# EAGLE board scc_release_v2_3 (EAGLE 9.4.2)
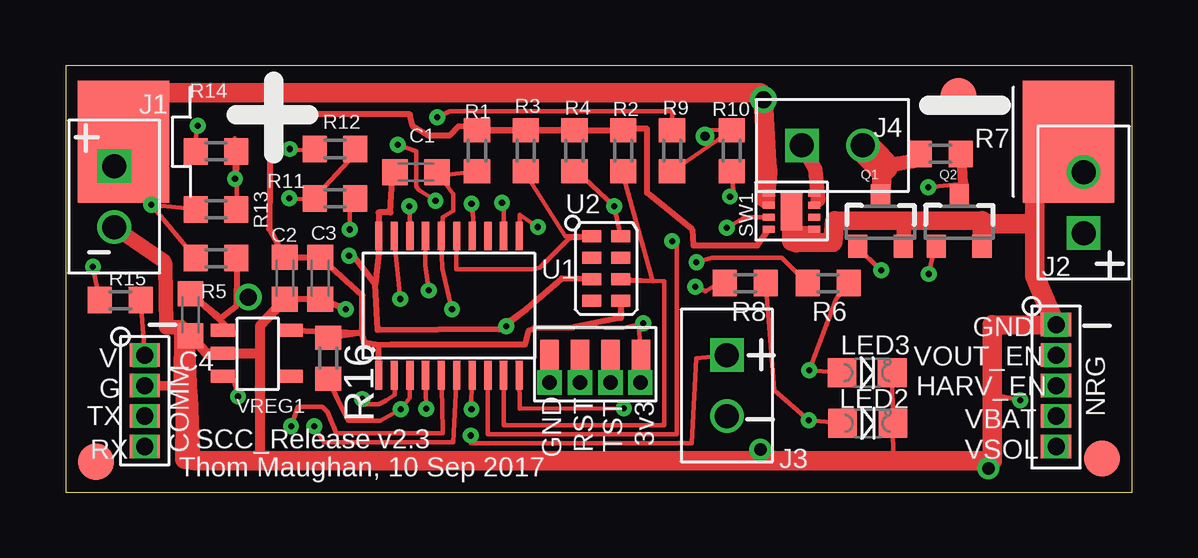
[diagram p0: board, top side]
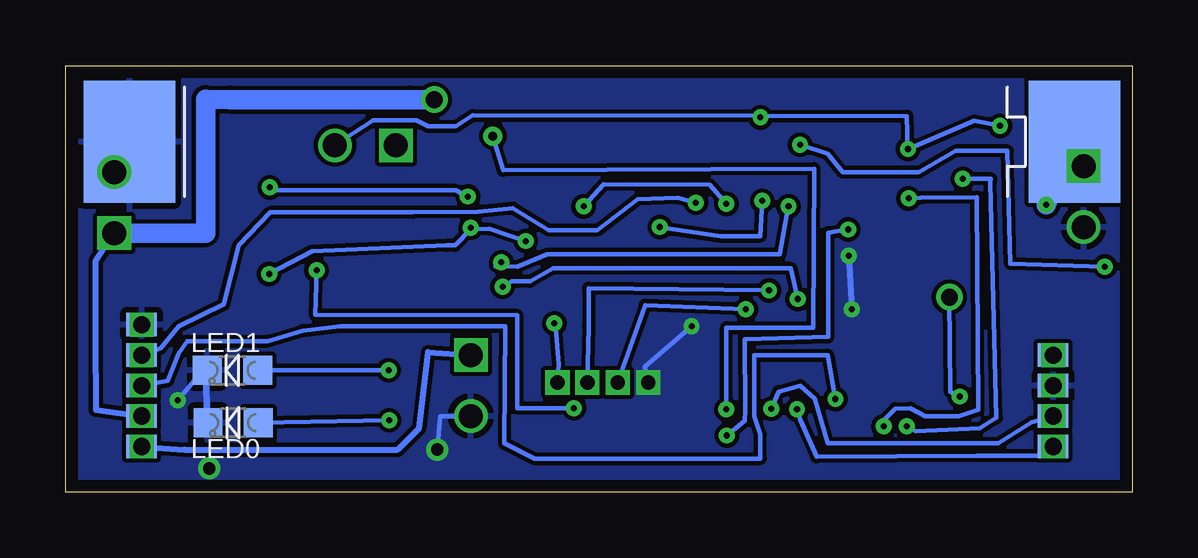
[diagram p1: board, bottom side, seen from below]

Size 44.45 x 17.78 mm. Coordinates in mm from the lower left corner, seen from the top.
Outline: 0,0 44.45,0 44.45,17.78 0,17.78 0,0
Copper layers (1*16): Top 0.035mm / dielectric 1.5mm / Bottom 0.035mm
Design rules "default *": minimum track width 7mil, minimum drill 8mil, track to track 7mil, track to pad 7mil, pad to pad 7mil, via to via 7mil, smd to smd 7mil, copper to edge 20mil, drill to drill 7mil, minimum pad ring 5mil, minimum via ring 8mil, stop-mask expansion 4mil, vias tented up to drill 11mil, thermal gap 10mil

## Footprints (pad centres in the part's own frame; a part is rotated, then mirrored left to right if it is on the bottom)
BAT_10440 = smd 3.81 x 5.08: P$1 0.508,4.572; P$2 39.878,4.572
C0603K = smd 1.05 x 1.08: 1 -0.875,0; 2 0.875,0
CON_1X4_050 = drill 0.711 pad 0.965 square: P$1 0,1.905; P$2 0,0.635; P$3 0,-0.635; P$4 0,-1.905 | smd 1.27 x 0.965: P$5 0,1.905; P$6 0,0.635; P$7 0,-0.635; P$8 0,-1.905 | smd 1.27 x 0.965 bottom: P$9 0,1.905; P$10 0,0.635; P$11 0,-0.635; P$12 0,-1.905
EMU_MSP_SPYBYWIRE_4_050 = smd 1.524 x 0.762: P1_3V3 0,1.905; P2_TST 0,0.635; P3_RST* 0,-0.635; P4_GND 0,-1.905
CON_1X2_0_1 = drill 1 square: P$1 0,1.27 | drill 1: P$2 0,-1.27
FIDUCIAL-1.5X3 = smd 1.5 x 1.5: 1 0,0
CHIPLED_0805 = smd 1.2 x 1.2: A 0,-1.05; C 0,1.05
CON_1X5_050 = drill 0.711 pad 0.965 square: P$1 0,2.54; P$2 0,1.27; P$3 0,0; P$4 0,-1.27; P$5 0,-2.54 | smd 1.27 x 0.965: P$6 0,2.54; P$7 0,1.27; P$8 0,0; P$9 0,-1.27; P$10 0,-2.54 | smd 1.27 x 0.965 bottom: P$11 0,2.54; P$12 0,1.27; P$13 0,0; P$14 0,-1.27; P$15 0,-2.54
SOT23-3 = smd 0.8 x 0.95: 1 -0.95,-1; 2 0.95,-1; 3 0,1.1
R0603 = smd 1 x 1.1: 1 -0.85,0; 2 0.85,0
TI_WSON8 = smd 0.5 x 0.28: P$1 -0.95,0.75; P$2 -0.95,0.25; P$3 -0.95,-0.25; P$4 -0.95,-0.75; P$5 0.95,-0.75; P$6 0.95,-0.25; P$7 0.95,0.25; P$8 0.95,0.75 | smd 0.9 x 1.6: P$9 0,0
PW20 = smd 0.3 x 1.2: 1 -2.925,-2.9; 2 -2.275,-2.9; 3 -1.625,-2.9; 4 -0.975,-2.9; 5 -0.325,-2.9; 6 0.325,-2.9; 7 0.975,-2.9; 8 1.625,-2.9; 9 2.275,-2.9; 10 2.925,-2.9; 11 2.925,2.9; 12 2.275,2.9; 13 1.625,2.9; 14 0.975,2.9; 15 0.325,2.9; 16 -0.325,2.9; 17 -0.975,2.9; 18 -1.625,2.9; 19 -2.275,2.9; 20 -2.925,2.9
M41T62_PKG = smd 0.8 x 0.5: P$1 -0.6,1.35; P$2 -0.6,0.45; P$3 -0.6,-0.45; P$4 -0.6,-1.35; P$5 0.6,-1.35; P$6 0.6,-0.45; P$7 0.6,0.45; P$8 0.6,1.35
SOT23-5 = smd 1 x 0.54: P$1 -1.431,0.95; P$2 -1.431,0; P$3 -1.431,-0.95; P$4 1.419,-0.95; P$5 1.419,0.95

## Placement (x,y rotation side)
BAT1  [BAT_10440]  42.29,10.03 0 bottom
BAT2  [BAT_10440]  42.29,19.18 180 top
C1  2.2 nF  [C0603K]  14.61,13.34 180 top
C2  10 uF  [C0603K]  9.14,8.92 270 top
C3  0.1 uF  [C0603K]  10.62,8.92 270 top
C4  10 uF  [C0603K]  5.21,7.39 270 top
COMM  [CON_1X4_050]  3.3,3.81 0 top
EMU1  spybywire  [EMU_MSP_SPYBYWIRE_4_050]  22.07,5.59 270 top
J1  [CON_1X2_0_1]  2.03,12.32 0 top
J2  [CON_1X2_0_1]  42.42,12.06 180 top
J3  Solar  [CON_1X2_0_1]  27.56,4.45 0 top
J4  RELEASE  [CON_1X2_0_1]  31.95,14.45 90 top
JP1  FIDUCIAL1.5X3  [FIDUCIAL-1.5X3]  1.27,1.27 0 top
JP2  FIDUCIAL1.5X3  [FIDUCIAL-1.5X3]  43.18,1.4 0 top
JP3  FIDUCIAL1.5X3  [FIDUCIAL-1.5X3]  37.21,16.51 0 top
LED0  GREEN  [CHIPLED_0805]  37.47,2.9 90 bottom
LED1  RED  [CHIPLED_0805]  37.49,5.08 90 bottom
LED2  GREEN  [CHIPLED_0805]  33.43,2.87 270 top
LED3  RED  [CHIPLED_0805]  33.4,4.98 270 top
NRG  [CON_1X5_050]  41.27,4.45 0 top
Q1  DMN2075U-7  [SOT23-3]  33.96,11.25 0 top
Q2  DMN2075U-7  [SOT23-3]  37.24,11.25 0 top
R1  47K  [R0603]  17.14,14.22 270 top
R2  1M  [R0603]  23.24,14.22 270 top
R3  10K  [R0603]  19.18,14.22 270 top
R4  10K  [R0603]  21.21,14.22 270 top
R5  10  [R0603]  6.27,9.75 0 top
R6  1K  [R0603]  31.78,8.71 0 top
R7  30  [R0603]  36.45,14.1 180 top
R8  1K  [R0603]  28.32,8.71 0 top
R9  10K  [R0603]  25.27,14.22 270 top
R10  10K  [R0603]  27.76,14.22 90 top
R11  100K  [R0603]  11.23,12.24 180 top
R12  100K  [R0603]  11.23,14.3 180 top
R13  100K  [R0603]  6.27,11.79 0 top
R14  100K  [R0603]  6.27,14.2 180 top
R15  100K  [R0603]  2.29,8 0 top
R16  1M  [R0603]  10.95,5.59 270 top
SW1  TPS22965N  [TI_WSON8]  30.25,11.71 0 top
U1  MSP430G2553  [PW20]  15.98,7.77 0 top
U2  M41T62  [M41T62_PKG]  22.53,9.32 0 top
VREG1  TPS78330  [SOT23-5]  7.98,5.79 0 top

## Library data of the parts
BAT1 BAT2 EMU1 SW1 = ti_thom
C1-C4 R1-R16 = resistor
COMM J1-J4 NRG Q1 Q2 VREG1 = thomz
JP1-JP3 = EM-shield-V1.0A
LED0 LED1-LED3 = led
U1 = TI_MSP430_v16
U2 = thomz_rtc

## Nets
ALARM*: R2.2 U1.9 U2.P$6
GND: BAT1.P$1 BAT2.P$1 C1.2 C2.2 C3.2 C4.2 COMM.P$2 COMM.P$6 COMM.P$10 EMU1.P4_GND J1.P$2 J2.P$2 J3.P$2 LED0.C LED1.C LED2.C LED3.C NRG.P$1 NRG.P$6 NRG.P$11 Q1.2 Q2.2 SW1.P$5 SW1.P$9 U1.20 U2.P$3 VREG1.P$2
HARVEST_EN#: NRG.P$3 NRG.P$8 NRG.P$13 U1.2
HI_REL_LO_CONT: Q2.1 SW1.P$3 U1.8
LED0: R8.1 U1.19
LED1: R6.1 U1.18
LO_REL: Q1.1 U1.10
N$1: LED1.A LED3.A R6.2
N$4: Q2.3 R7.1 R10.1
N$19: LED0.A LED2.A R8.2
RELEASE_HI: J4.P$1 SW1.P$7 SW1.P$8
RELEASE_LO: J4.P$2 Q1.3 R7.2 R9.1 R12.2 R14.2
RST*: C1.1 EMU1.P3_RST* R1.2 U1.16
RXD: COMM.P$4 COMM.P$8 COMM.P$12 R16.2 U1.3
SCL: R4.2 U1.14 U2.P$8
SDA: R3.2 U1.15 U2.P$1
TCK: EMU1.P2_TST U1.17
TXD: COMM.P$3 COMM.P$7 COMM.P$11 U1.4
VBAT: BAT1.P$2 BAT2.P$2 J1.P$1 J2.P$1 NRG.P$4 NRG.P$9 NRG.P$14 R5.1 R13.1 SW1.P$1 SW1.P$2
VBATMON: R13.2 R14.1 U1.5
VBUCK_OUT: COMM.P$1 COMM.P$5 COMM.P$9 R15.2
VCC: C2.1 C3.1 EMU1.P1_3V3 R1.1 R2.1 R3.1 R4.1 R16.1 SW1.P$4 U1.1 U2.P$5 VREG1.P$5
VCONTMON: R9.2 R10.2 U1.7
VIN: C4.1 R5.2 VREG1.P$1 VREG1.P$3
VOUT_ACT: R15.1 U1.11
VOUT_EN: NRG.P$2 NRG.P$7 NRG.P$12 U1.12
VSOL: J3.P$1 NRG.P$5 NRG.P$10 NRG.P$15 R11.1
VSOLMON: R11.2 R12.1 U1.6

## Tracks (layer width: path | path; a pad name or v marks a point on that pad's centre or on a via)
ALARM*
  Top 0.178: 23.19,13.32 24.46,8.79 23.38,8.81 | U2.P$6 24.94,8.8 24.94,2.79 18.26,2.79 U1.9
  Top 0.254: R2.2 23.19,13.32 | 23.38,8.81 U2.P$6
GND  (via drill 0.25, 0.51, 0.6)
  Top 0.178: EMU1.P4_GND v20.17,4.57 | v18.36,6.91 19.21,7.57 19.21,7.63 | BAT2.P$1 J2.P$2 | VREG1.P$2 8.03,5.66 | 27.53,1.32 v28.96,1.78 | v39.78,3.83 38.61,4.09 | LED3.C LED2.C 34.49,1.32
  Top 0.254: 12.9,8.66 13.06,9.99 13.08,10.67 U1.20 13.05,11.66 13.54,11.66 13.61,13.06 13.77,13.31 C1.2 | U2.P$3 20.68,8.9 19.21,7.63 18.06,6.78 13.01,6.76 12.9,8.66 | SW1.P$5 30.25,10.96 | C2.2 C3.2 v11.68,7.62 | 12.9,8.66 11.94,9.91 v11.81,9.86
  Top 0.406: 30.25,10.96 SW1.P$9 | 5.41,1.32 5.31,4.04 C4.2 5.89,5.77 VREG1.P$2 8.03,5.79 | C2.2 8.1,6.93 8.1,1.32 | COMM.P$6 4.79,4.46
  Top 0.61: Q1.2 34.92,10.3 34.92,11.18 35.76,11.3 | 30.45,10.39 30.71,10.72 30.25,10.46 | Q2.2 38.2,10.25 | J1.P$2 4.06,9.65 | 4.79,4.46 4.83,6.88 4.19,6.88 4.17,9.5 4.09,9.65
  Top 0.762: 32.05,11.3 35.76,11.3 38.2,11.3
  Top 0.813: 32.05,11.3 31.98,10.41 30.45,10.39 | 30.25,10.46 30.25,10.96 | 38.2,10.25 38.2,11.3 | Q2.2 38.23,11.18 40.39,11.18 | 40.39,11.18 40.39,13.21 J2.P$2 | 40.39,11.18 40.39,9.02 41.2,7.09 NRG.P$6 41.25,6.96 38.61,6.99 38.61,4.09 38.61,1.32 34.49,1.32 27.53,1.32 8.1,1.32 5.41,1.32 4.98,1.37 5,4.88
  Bottom 0.178: v20.17,4.57 20.32,5.23 v18.36,6.91 | 38.51,5.08 LED1.C LED0.C 38.61,2.85 38.63,5.18 v39.78,3.83 | BAT2.P$1 J2.P$2 | v28.96,1.78 28.83,3.17 J3.P$2
  Bottom 0.254: v11.81,9.86 v11.68,7.62
  other vias: 38.46,0.99
  pour Bottom: -0.13,17.88 -0.13,-0.38 44.86,-0.38 44.86,18.14 0.23,18.14 0.23,18.08
HARVEST_EN#  (via drill 0.25)
  Top 0.178: U1.2 13.72,4.06 13.34,3.81 13.06,3.66 12.42,3.66 v12.37,3.89
  Bottom 0.178: v12.37,3.89 12.7,5.71 15.75,5.71 15.75,3.17 15.49,2.41 15.49,1.4 24.89,1.4 26.16,2.03 26.14,6.91 32.99,6.91 34.57,6.73 36.02,6.3 39.37,6.3 39.73,5.79 40.18,4.65 NRG.P$13
HI_REL_LO_CONT  (via drill 0.25)
  Top 0.178: SW1.P$3 28.47,11.46 28.25,11.41 v27.56,11.02 | v35.97,9.09 36.26,10.41 Q2.1 | v25.27,10.46 25.38,10.46 25.48,10.39 25.48,9.14 25.48,2.41 17.6,2.41 17.6,3.53 U1.8
  Bottom 0.178: 27.56,10.96 28.22,10.29 28.57,10.29 34.16,10.03 v35.97,9.09 | v25.27,10.46 26.8,10.97 27.56,10.96 | 27.56,10.96 v27.56,11.02
LED0  (via drill 0.25)
  Top 0.178: U1.19 13.72,10.31 v13.95,8.05 | v26.24,8.56 26.67,8.38 27.3,8.76 R8.1
  Bottom 0.178: v13.95,8.05 14.22,9.32 24.13,9.32 25.09,8.79 25.63,8.79 25.86,8.79 v26.24,8.56
LED1  (via drill 0.25)
  Top 0.178: v14.33,11.91 14.38,10.7 U1.18 | R6.1 30.23,9.4 29.84,9.78 26.92,9.78 v26.29,9.58
  Bottom 0.178: v14.33,11.91 14.68,9.91 24.38,9.91 25.63,9.4 26.54,9.42 v26.29,9.58
LO_REL  (via drill 0.25)
  Top 0.178: v23.27,3.5 18.93,3.48 U1.10 | v33.98,9.25 33.29,9.91 Q1.1
  Bottom 0.178: v23.27,3.5 25.63,3.5 25.63,7.37 34.04,7.39 v33.98,9.25
N$1  (via drill 0.25)
  Top 0.178: R6.2 32.11,8.05 v30.99,5.08 LED3.A
  Bottom 0.178: v30.99,5.08 LED1.A
N$4  (via drill 0.25)
  Top 0.178: R10.1 27.81,12.57 27.69,12.45 v27.69,12.32 | v35.94,12.7 37.41,12.85
  Top 0.406: Q2.3 37.41,12.85 37.34,13.87 37.32,13.82 R7.1
  Bottom 0.178: v27.69,12.32 28.19,12.57 35.69,12.57 v35.94,12.7
N$19  (via drill 0.25)
  Top 0.178: R8.2 29.54,4.24 v30.96,3 LED2.A
  Bottom 0.178: v30.96,3 LED0.A
RELEASE_HI
  Top 0.305: 31.37,12.19 SW1.P$7 SW1.P$8
  Top 0.61: J4.P$1 31.24,13.46 31.37,12.19
RELEASE_LO  (via drill 0.25)
  Top 0.178: R12.2 9.98,14.25 v9.35,14.3 | v5.51,15.27 5.3,13.99 R14.2 | v15.49,15.62 16,15.88 25.27,15.88 R9.1
  Top 0.61: 34.06,13.59 35.31,13.79 35.47,13.95 R7.2
  Top 0.813: 34.06,13.59 Q1.3
  Top 1.27: 34.06,13.59 J4.P$2
  Bottom 0.178: v5.51,15.27 6.58,15.47 v9.35,14.3 9.4,15.67 15.75,15.68 | 15.75,15.68 27.48,15.7 28.19,15.24 29.34,15.24 29.84,15.49 31.62,15.49 J4.P$2 | v15.49,15.62 15.75,15.68
RST*  (via drill 0.25, 0.6)
  Top 0.178: 15.65,10.41 15.65,10.62 15.72,11.46 16.15,11.73 16.15,12.42 C1.1 15.75,13.21 R1.2 | 15.65,10.41 15.7,9.32 v16.1,7.62 | v21.44,4.57 21.31,5.33 EMU1.P3_RST* | U1.16 15.65,10.41
  Top 0.254: 17.2,13.31 R1.2
  Bottom 0.178: v16.1,7.62 20.3,7.8 v21.44,4.57
RXD  (via drill 0.25)
  Top 0.178: U1.3 14.35,5.18 14.35,3.94 v13.97,3.45 13.11,2.97 11.79,2.97 11.35,3.86 R16.2
  Bottom 0.178: v13.97,3.45 13.84,3.02 13.16,1.47 6.48,1.52 3.81,1.52 COMM.P$8
SCL  (via drill 0.25)
  Top 0.178: U1.14 16.99,11.43 v16.92,12.01 | R4.2 20.95,13.72 v22.86,11.91 U2.P$8
  Top 0.254: v16.92,12.01 16.99,12.01
  Bottom 0.178: v16.92,12.01 17.6,12.8 22.02,12.83 v22.86,11.91
SDA
  Top 0.178: 21.04,10.62 19.76,9.35 19.43,9.3 16.28,9.3 16.31,10.75 U1.15 | U2.P$1 20.83,10.67 19.05,13.46 R3.2
  Top 0.254: 21.04,10.62 U2.P$1
TCK  (via drill 0.25, 0.6)
  Top 0.178: v22.71,4.57 22.61,5.82 EMU1.P2_TST | U1.17 14.99,9.45 v15.14,8.41
  Bottom 0.178: v15.14,8.41 22.66,8.51 22.66,6.99 22.66,6.88 v22.71,4.57
TXD  (via drill 0.25)
  Top 0.178: U1.4 14.99,5.05 v15.04,3.48
  Bottom 0.178: v15.04,3.48 14.73,4.19 13.84,4.45 13.23,3.89 12.7,2.03 5.59,2.03 4.19,2.92 COMM.P$7
VBAT  (via drill 0.25, 0.7)
  Top 0.178: R5.1 v3.58,11.97 | R13.1 v3.58,11.97 | v3.58,11.97 J1.P$1 BAT2.P$2 | 29.16,12.24 SW1.P$2
  Top 0.254: SW1.P$2 29.11,12.29
  Top 0.406: 29.11,12.29 29.11,12.95 | 29.3,12.45 SW1.P$1 29.01,12.74 29.16,12.24
  Top 0.813: 29.16,12.24 29.26,13.36 29.21,13.72 v29.08,16.36 | v29.08,16.36 28.96,16.64 | 28.96,16.64 2.16,16.64 J1.P$1 | v29.08,16.36 28.96,16.64
  Bottom 0.254: J2.P$1 43.18,9.65 43.18,4.95 43.18,3.43 NRG.P$4
  Bottom 0.813: BAT2.P$2 v3.58,11.97 | J2.P$1 38.61,10.79 38.61,16.38 37.59,16.36 30.1,16.36 v29.08,16.36
VBATMON  (via drill 0.25)
  Top 0.178: R13.2 7.16,13.97 | 7.16,13.97 7.19,14.28 R14.1 | v9.4,2.74 9.68,3.56 10.69,3.56 10.92,3.33 11.28,2.46 15.72,2.46 15.7,3.63 15.65,4.8 U1.5 | v7.06,13.06 7.06,14.76 7.16,13.97
  Bottom 0.178: v7.06,13.06 5.89,13.06 5.92,12.9 5.66,3.1 6.35,2.67 9.02,2.54 v9.4,2.74
VBUCK_OUT
  Top 0.178: COMM.P$9 R15.2
VCC  (via drill 0.25, 0.6)
  Top 0.178: EMU1.P1_3V3 23.9,6.73 EMU1.P1_3V3 | 21.18,6.88 22.45,6.86 23.27,6.86 23.65,6.93 v24.08,7.04 | EMU1.P1_3V3 v23.95,4.57 | U1.1 13.06,5.56
  Top 0.254: 13.06,4.82 13.06,5.56 13.06,6.12 | 13.06,6.12 12.45,6.22 12.37,6.64 | VREG1.P$5 12.37,6.64 | 12.37,6.64 12.37,8.2 11.05,9.4 C3.1 C2.1 8.48,10.97 8.53,15.21 8.89,15.75 14.35,15.75 14.48,15.24 15.11,14.86 16,14.86 16.38,15.24 17.5,15.21 R1.1 | R1.1 R3.1 R4.1 | R4.1 R2.1 23.39,15.14 24.23,15.14 24.23,12.47 26.11,10.95 26.16,10.29 28.83,10.29 SW1.P$4 29.29,10.96 | U2.P$5 23.14,7.26 21.18,6.88 19.56,6.86 19.3,6.73 19.15,6.15 13.56,6.15 13.06,6.12 | R4.1 R1.1 | 12.37,6.64 R16.1
  Bottom 0.178: v23.95,4.57 23.9,5.31 24.03,6.86 24.13,6.96 v24.08,7.04
VCONTMON  (via drill 0.25, 0.38)
  Top 0.178: U1.7 16.92,3.79 v16.92,3.45 | R9.2 R10.2 26.68,15.1 v26.64,14.83
  Bottom 0.178: v16.92,3.45 16.92,6.86 13.28,6.86 13.26,13.49 26.21,13.41 v26.64,14.83
VIN  (via drill 0.25, 0.7)
  Top 0.178: v7.62,8.13 7.11,7.75 | VREG1.P$3 7.01,4.66 v7.19,3.99
  Top 0.254: VREG1.P$1 7,6.64 C4.1 6.48,7.24 7.11,7.75 7.13,9.25 R5.2
  Bottom 0.178: 8,7.87 v7.62,8.13 7.59,4.19 v7.19,3.99
VOUT_ACT  (via drill 0.25)
  Top 0.178: R15.1 v1.14,9.4 | U1.11 18.92,11.56 v19.68,11.05 | v15.42,12.14 14.73,12.57 14.61,12.72 14.61,14.2 v13.84,14.48
  Bottom 0.178: v1.14,9.4 5.08,9.53 5.21,14.22 7.37,14.22 8.89,13.34 12.06,13.34 12.7,14.1 v13.84,14.48 | v19.68,11.05 17.14,10.67 15.49,10.67 v15.42,12.14
VOUT_EN  (via drill 0.25)
  Top 0.178: U1.12 18.26,11.89 v18.19,12.06
  Bottom 0.178: v18.19,12.06 18.95,12.27 20.6,12.22 22.3,10.92 24.31,10.92 25.81,11.84 27.25,11.68 29.97,11.66 35.92,11.66 37.24,10.29 37.85,7.82 39.73,6.91 40.49,5.99 NRG.P$12
VSOL  (via drill 0.25)
  Top 0.178: R11.1 11.86,11.89 11.84,11.66 v11.84,10.95 | v16.89,2.36 16.82,2.39 16.89,2.03 26.09,2.03 26.29,5.59 J3.P$1
  Bottom 0.178: v16.89,2.36 16.15,2.97 16.13,3.43 16.15,6.38 12.68,6.48 12.68,10.82 v11.84,10.95 | NRG.P$5 41.27,1.96
  Bottom 0.254: NRG.P$5 39.5,1.78 30.61,1.78 29.72,2.67 29.34,5.84 J3.P$1
VSOLMON  (via drill 0.25)
  Top 0.178: v10.36,2.74 10.77,2.08 16.15,2.08 16.28,4.5 U1.6 | v9.32,12.24 10.3,12.19 | R11.2 10.3,12.19 | 10.3,12.19 11.8,13.82 R12.1
  Bottom 0.178: v10.36,2.74 10.31,3.05 9.88,3.48 9.25,3.5 8.64,3.17 7.24,3.17 6.43,3.43 6.48,12.29 8.81,12.27 v9.32,12.24

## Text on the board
tPlace: GND | V | VOUT_EN | G | HARV_EN | TX | VBAT | SCC_Release v2.3 | RST | TST | 3v3 | RX | Thom Maughan, 10 Sep 2017 | GND | VSOL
